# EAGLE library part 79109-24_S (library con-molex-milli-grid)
RECEPTACAL
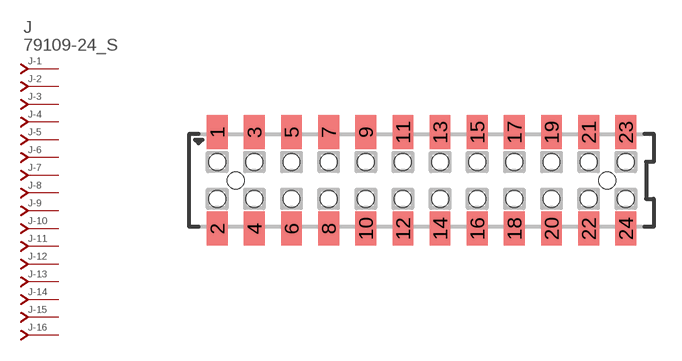
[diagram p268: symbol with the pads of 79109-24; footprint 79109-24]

Designator prefix J; gates -1=J-NV -2=J-N -3=J-N -4=J-N -5=J-N -6=J-N -7=J-N -8=J-N -9=J-N -10=J-N -11=J-N -12=J-N -13=J-N -14=J-N -15=J-N -16=J-N -17=J-N -18=J-N -19=J-N -20=J-N -21=J-N -22=J-N -23=J-N -24=J-N

## 79109-24_S  [79109-24]
1  -1:J  pas
2  -2:J  pas
3  -3:J  pas
4  -4:J  pas
5  -5:J  pas
6  -6:J  pas
7  -7:J  pas
8  -8:J  pas
9  -9:J  pas
10  -10:J  pas
11  -11:J  pas
12  -12:J  pas
13  -13:J  pas
14  -14:J  pas
15  -15:J  pas
16  -16:J  pas
17  -17:J  pas
18  -18:J  pas
19  -19:J  pas
20  -20:J  pas
21  -21:J  pas
22  -22:J  pas
23  -23:J  pas
24  -24:J  pas

## Footprint 79109-24 (pad centres in mm)
RECEPTACAL SMD Dual Row, Vertical, Pass-Thru
smd 1.12 x 1.83: 1 -11,2.6; 2 -11,-2.6; 3 -9,2.6; 4 -9,-2.6; 5 -7,2.6; 6 -7,-2.6; 7 -5,2.6; 8 -5,-2.6; 9 -3,2.6; 10 -3,-2.6; 11 -1,2.6; 12 -1,-2.6; 13 1,2.6; 14 1,-2.6; 15 3,2.6; 16 3,-2.6; 17 5,2.6; 18 5,-2.6; 19 7,2.6; 20 7,-2.6; 21 9,2.6; 22 9,-2.6; 23 11,2.6; 24 11,-2.6
hole 0.914 at -10,0
hole 0.914 at -11,1
hole 0.914 at -11,-1
hole 0.914 at -9,-1
hole 0.914 at -9,1
hole 0.914 at -7,-1
hole 0.914 at -7,1
hole 0.914 at 10,0
hole 0.914 at -5,1
hole 0.914 at -5,-1
hole 0.914 at -3,1
hole 0.914 at -3,-1
hole 0.914 at -1,1
hole 0.914 at -1,-1
hole 0.914 at 1,1
hole 0.914 at 1,-1
hole 0.914 at 3,-1
hole 0.914 at 3,1
hole 0.914 at 5,1
hole 0.914 at 5,-1
hole 0.914 at 7,1
hole 0.914 at 7,-1
hole 0.914 at 9,1
hole 0.914 at 9,-1
hole 0.914 at 11,-1
hole 0.914 at 11,1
